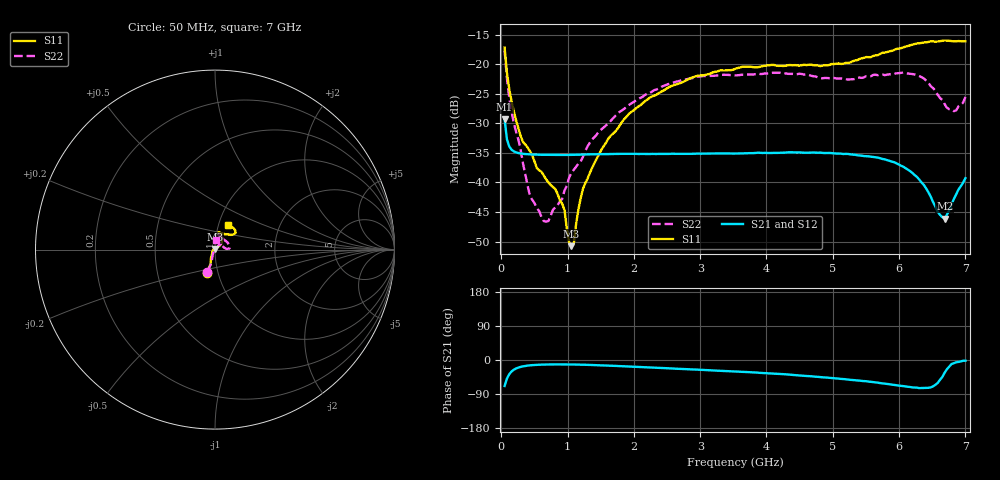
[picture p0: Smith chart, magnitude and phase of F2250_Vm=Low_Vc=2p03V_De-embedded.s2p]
! Integrated Device Technology
! Corporate Headquarters
! 6024 Silver Creek Valley Road
! San Jose, CA 95138  USA
! Phone:  1-408-284-8200
! Toll Free:  1-800-223-1366
! Webpage:  http://www.idt.com/
! Timing and RF Division
! 515 Groton Road, Suite 102
! Westford, MA 01886-6024
! Device:  F2250
! Description: Voltage Variable RF Attenuator
! Frequency:  50.0 -  6000.00 MHz
! Package:  3x3 mm Thin QFN Plastic Package: 16 pin
! Ports:  2 RF, 3 DC
!  Pin  1  = GND
!  Pin  2  = NC
!  Pin  3  = RF1  = Port 1
!  Pin  4  = NC
!  Pin  5  = GND
!  Pin  6  = GND
!  Pin  7  = GND
!  Pin  8  = GND
!  Pin  9  = NC
!  Pin 10  = RF2  = Port 2
!  Pin 11  = NC
!  Pin 12  = GND
!  Pin 13  = GND
!  Pin 14  = VCNTRL
!  Pin 15  = VDD
!  Pin 16  = VMODE
! Vcntrl:  2.030 Volts
! Vmode:  +0.000 Volts
! Vdd:  +3.30  Volts
! Current:  1.180 mA
! Data:  The device was measured on a the F2250 evaluation board which has
!  individual transmission lines to the RF pins.  Data was collected
!  using a calibrated network analyzer.  The evaluation board was
!  de-embedded using a TRL calibration technique.
!  The reference plane is the edge of the package pin.
! Misc:  SN 10
!  Action Tracker AT0258
! Date Measured:  2014-11-26
! Date:  2015-10-15  MJV
! Note:
!  Integrated Device Technology supplies this data as a sample of measured
!  data at the package pin for this product.  Your particular data for this
!  product may vary.
!  Data was taken at 25 degrees C.
!  Integrated Device Technology reserves the right to change this data at anytime.
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# GHz S dB R 50
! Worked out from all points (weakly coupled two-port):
!   201 points, 50 MHz to 7 GHz, reference 50 ohm
!   highest |S21| = -29.29 dB at 50 MHz (marker M1); lowest = -46.1 dB at 6.687 GHz (marker M2)
!   lowest |S11| = -50.8 dB at 1.058 GHz (marker M3), VSWR 1.01, Z = 49.8 + j0.241 ohm
!   |S11| at or under -10 dB: start of sweep to end of sweep
!   |S22| runs from -46.6 to -17.7 dB; largest |S21 - S12| = 6.4e-05
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0.05  -17.18 -108.6  -29.29 -68.5  -29.29 -68.5  -17.72 -108.9
0.08475  -21.44 -107.4  -32.69 -49.2  -32.69 -49.2  -22.37 -104.9
0.1195  -24.19 -111.8  -33.91 -37.5  -33.91 -37.6  -25.65 -108.1
0.29325  -32.21 -127.7  -35.10 -18.1  -35.10 -18.1  -34.56 -117.4
0.43225  -34.71 -144.6  -35.25 -14.1  -35.26 -14.1  -42.27 -148.5
0.606  -38.19 -161.0  -35.32 -12.2  -35.32 -12.2  -45.84 162.6
0.71025  -39.97 -168.4  -35.34 -11.8  -35.34 -11.8  -46.53 127.9
0.91875  -43.60 158.0  -35.35 -11.7  -35.35 -11.7  -42.76 88.4
1.023  -50.13 143.7  -35.34 -11.8  -35.34 -11.8  -39.19 75.0
1.05775  -50.78 123.3  -35.34 -11.8  -35.34 -11.8  -38.34 71.6
1.0925  -50.47 89.6  -35.33 -11.9  -35.33 -11.9  -37.87 67.4
1.162  -44.63 56.6  -35.31 -12.1  -35.31 -12.1  -36.82 57.9
1.2315  -41.08 44.1  -35.28 -12.4  -35.28 -12.4  -35.68 51.7
1.6485  -32.10 41.9  -35.20 -15.0  -35.20 -15.0  -29.61 47.8
2.37825  -24.88 47.4  -35.17 -20.8  -35.17 -20.8  -24.08 48.2
3.525  -20.81 72.5  -35.11 -30.3  -35.11 -30.4  -21.89 70.3
4.7065  -20.17 72.3  -34.94 -43.4  -34.93 -43.5  -22.03 69.7
5.85325  -17.82 40.4  -36.34 -64.0  -36.34 -64.0  -21.71 18.3
6.33975  -16.41 41.0  -40.01 -73.9  -40.02 -74.0  -22.19 4.2
6.68725  -15.99 48.8  -46.12 -33.3  -46.11 -33.0  -26.76 24.5
6.861  -16.12 55.1  -42.01 -6.0  -41.98 -6.0  -27.81 58.5
7  -16.12 63.2  -39.28 -1.9  -39.24 -2.0  -25.55 86.6
